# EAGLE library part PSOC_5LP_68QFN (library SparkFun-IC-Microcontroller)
PSoC5LP 68-QFN package CY8C5868LTI-LP039 PSOC 5LP 256K/64K/2K 80MHz Datasheet SparkFun Products FreeSoC2 Development Board - PSoC5LP (DEV-13229) -- Involved with change to new unposted revision
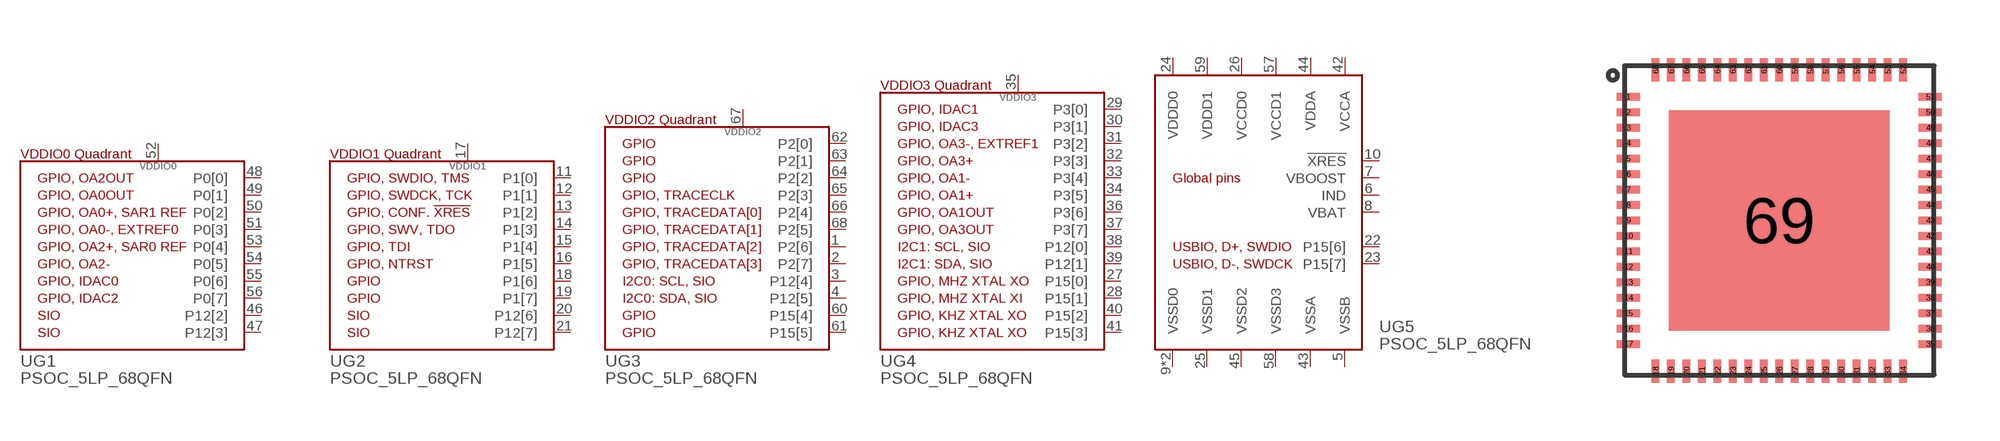
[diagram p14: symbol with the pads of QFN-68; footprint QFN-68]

Designator prefix U; gates G1=CY8C58LP_68QFN_VDDIO0 G2=CY8C58LP_68QFN_VDDIO1 G3=CY8C58LP_68QFN_VDDIO2 G4=CY8C58LP_68QFN_VDDIO3 G5=CY8C58LP_68QFN_VGLOBAL

## PSOC_5LP_68QFN (PROD_ID: IC-12391; VALUE: CY8C5868LTI-LP039)  [QFN-68]
1  G3:P2[6]
2  G3:P2[7]
3  G3:P12[4]
4  G3:P12[5]
5  G5:VSSB
6  G5:IND
7  G5:VBOOST
8  G5:VBAT
9  G5:VSSD0
10  G5:!XRES
11  G2:P1[0]
12  G2:P1[1]
13  G2:P1[2]
14  G2:P1[3]
15  G2:P1[4]
16  G2:P1[5]
17  G2:VDDIO1
18  G2:P1[6]
19  G2:P1[7]
20  G2:P12[6]
21  G2:P12[7]
22  G5:P15[6]
23  G5:P15[7]
24  G5:VDDD0
25  G5:VSSD1
26  G5:VCCD0
27  G4:P15[0]
28  G4:P15[1]
29  G4:P3[0]
30  G4:P3[1]
31  G4:P3[2]
32  G4:P3[3]
33  G4:P3[4]
34  G4:P3[5]
35  G4:VDDIO3
36  G4:P3[6]
37  G4:P3[7]
38  G4:P12[0]
39  G4:P12[1]
40  G4:P15[2]
41  G4:P15[3]
42  G5:VCCA
43  G5:VSSA
44  G5:VDDA
45  G5:VSSD2
46  G1:P12[2]
47  G1:P12[3]
48  G1:P0[0]
49  G1:P0[1]
50  G1:P0[2]
51  G1:P0[3]
52  G1:VDDIO0
53  G1:P0[4]
54  G1:P0[5]
55  G1:P0[6]
56  G1:P0[7]
57  G5:VCCD1
58  G5:VSSD3
59  G5:VDDD1
60  G3:P15[4]
61  G3:P15[5]
62  G3:P2[0]
63  G3:P2[1]
64  G3:P2[2]
65  G3:P2[3]
66  G3:P2[4]
67  G3:VDDIO2
68  G3:P2[5]
69  G5:VSSD0

## Footprint QFN-68 (pad centres in mm)
smd 0.6 x 0.2: 1 -3.9,3.2; 2 -3.9,2.8; 3 -3.9,2.4; 4 -3.9,2; 5 -3.9,1.6; 6 -3.9,1.2; 7 -3.9,0.8; 8 -3.9,0.4; 9 -3.9,0; 10 -3.9,-0.4; 11 -3.9,-0.8; 12 -3.9,-1.2; 13 -3.9,-1.6; 14 -3.9,-2; 15 -3.9,-2.4; 16 -3.9,-2.8; 17 -3.9,-3.2; 35 3.9,-3.2; 36 3.9,-2.8; 37 3.9,-2.4; 38 3.9,-2; 39 3.9,-1.6; 40 3.9,-1.2; 41 3.9,-0.8; 42 3.9,-0.4; 43 3.9,0; 44 3.9,0.4; 45 3.9,0.8; 46 3.9,1.2; 47 3.9,1.6; 48 3.9,2; 49 3.9,2.4; 50 3.9,2.8; 51 3.9,3.2
smd 0.2 x 0.6: 18 -3.2,-3.9; 19 -2.8,-3.9; 20 -2.4,-3.9; 21 -2,-3.9; 22 -1.6,-3.9; 23 -1.2,-3.9; 24 -0.8,-3.9; 25 -0.4,-3.9; 26 0,-3.9; 27 0.4,-3.9; 28 0.8,-3.9; 29 1.2,-3.9; 30 1.6,-3.9; 31 2,-3.9; 32 2.4,-3.9; 33 2.8,-3.9; 34 3.2,-3.9; 52 3.2,3.9; 53 2.8,3.9; 54 2.4,3.9; 55 2,3.9; 56 1.6,3.9; 57 1.2,3.9; 58 0.8,3.9; 59 0.4,3.9; 60 0,3.9; 61 -0.4,3.9; 62 -0.8,3.9; 63 -1.2,3.9; 64 -1.6,3.9; 65 -2,3.9; 66 -2.4,3.9; 67 -2.8,3.9; 68 -3.2,3.9
smd 5.7 x 5.7: 69 0,0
